PROGRAM CORRIDOR
VAR	
	fbLight1: FB_Light;
	fbLight2: FB_Light;	
END_VAR
VAR_OUTPUT
	rTemperature: LREAL;
END_VAR

// Light 1
fbLight1(bOn:= , bOff:= , bToggle:= GVL.I_bTerm1_Var7, bLight=> GVL.Q_bTerm3_Var5);

// Light 2
fbLight2(bOn:= , bOff:= , bToggle:= GVL.I_bTerm1_Var8, bLight=> GVL.Q_bTerm3_Var6);

// Temperature
rTemperature := INT_TO_LREAL(GVL.I_nTerm5_Var4) / 10;

END_PROGRAM
